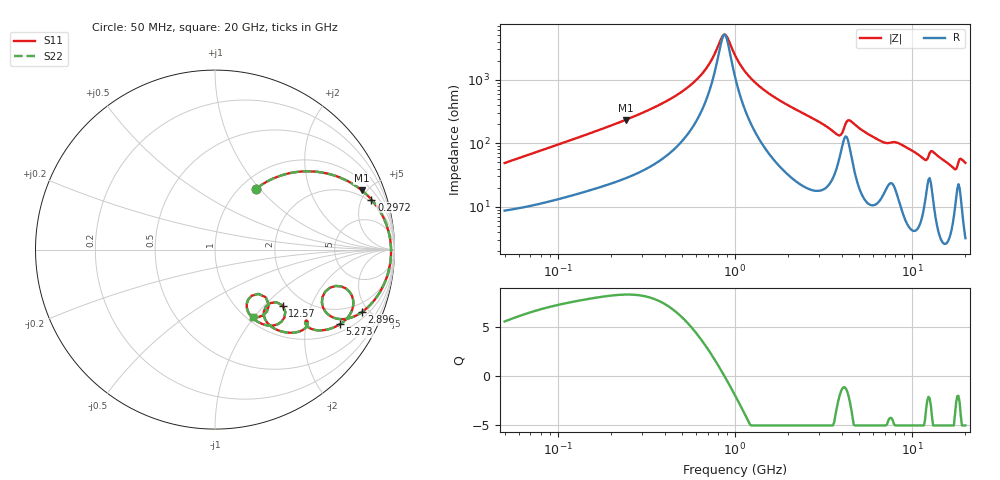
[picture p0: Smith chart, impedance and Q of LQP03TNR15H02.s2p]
!Murata Part Number: LQP03TNR15H02
!These Parameters are Measured in Series Mode Connection
!  o--[Z]--o
!Port1  Port2
!  o-------o
!Freq. Start=50[MHz] Stop=20[GHz], 401[Steps]
# Hz S RI R 50
!Freq.(Hz) S11(Real) S11(Imag) S21(Real) S21(Imag) S12(Real) S12(Imag) S22(Real) S22(Imag)
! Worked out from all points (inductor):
!   401 points, 50 MHz to 20 GHz, reference 50 ohm
!   read as one part in series: L = 151 nH near 51.52 MHz
!   highest Q = 8.25 at 241 MHz (marker M1), where L = 153 nH
!   self-resonance near 860.9 MHz
!   S11 on the Smith chart (normalised r, x): 50 MHz: 1.17, +0.96; 297.2 MHz: 1.73, +5.91; 2.896 GHz: 1.36, -4.53; 5.273 GHz: 1.29, -3.13; 12.57 GHz: 1.57, -1.29; 20 GHz: 1.06, -0.98
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5e7  0.2304 0.3403  0.7696 -0.3403  0.7696 -0.3403  0.2304 0.3403
1.364002e8  0.6106 0.4269  0.3894 -0.4269  0.3894 -0.4269  0.6106 0.4269
2.409965e8  0.8169 0.3308  0.1831 -0.3308  0.1831 -0.3308  0.8169 0.3308
2.972233e8  0.8712 0.2791  0.1288 -0.2791  0.1288 -0.2791  0.8712 0.2791
3.721004e8  0.9154 0.2202  0.0846 -0.2202  0.0846 -0.2202  0.9154 0.2202
6.285508e8  0.9713 0.083  0.0287 -0.083  0.0287 -0.083  0.9713 0.083
8.608917e8  0.9809 0.00315  0.0191 -0.00315  0.0191 -0.00315  0.9809 0.00315
1e9  0.9803 -0.0351  0.0197 0.0351  0.0197 0.0351  0.9803 -0.0351
1.411297e9  0.9653 -0.1267  0.0347 0.1267  0.0347 0.1267  0.9653 -0.1267
2.728004e9  0.8437 -0.3283  0.1563 0.3283  0.1563 0.3283  0.8437 -0.3283
2.896447e9  0.8195 -0.3474  0.1805 0.3474  0.1805 0.3474  0.8195 -0.3474
3.736399e9  0.6276 -0.3591  0.3724 0.3591  0.3724 0.3591  0.6276 -0.3591
4.212059e9  0.702 -0.2045  0.298 0.2045  0.298 0.2045  0.702 -0.2045
4.539627e9  0.7709 -0.2983  0.2291 0.2983  0.2291 0.2983  0.7709 -0.2983
5.273168e9  0.696 -0.4162  0.304 0.4162  0.304 0.4162  0.696 -0.4162
7.442007e9  0.5047 -0.3972  0.4953 0.3972  0.4953 0.3972  0.5047 -0.3972
9.457416e9  0.4161 -0.4631  0.5839 0.4631  0.5839 0.4631  0.4161 -0.4631
1.149051e10  0.2784 -0.3869  0.7216 0.3869  0.7216 0.3869  0.2784 -0.3869
1.257102e10  0.3773 -0.3124  0.6227 0.3124  0.6227 0.3124  0.3773 -0.3124
1.417136e10  0.2836 -0.4207  0.7164 0.4207  0.7164 0.4207  0.2836 -0.4207
1.747767e10  0.1841 -0.2796  0.8159 0.2796  0.8159 0.2796  0.1841 -0.2796
2e10  0.2093 -0.3755  0.7907 0.3755  0.7907 0.3755  0.2093 -0.3755
